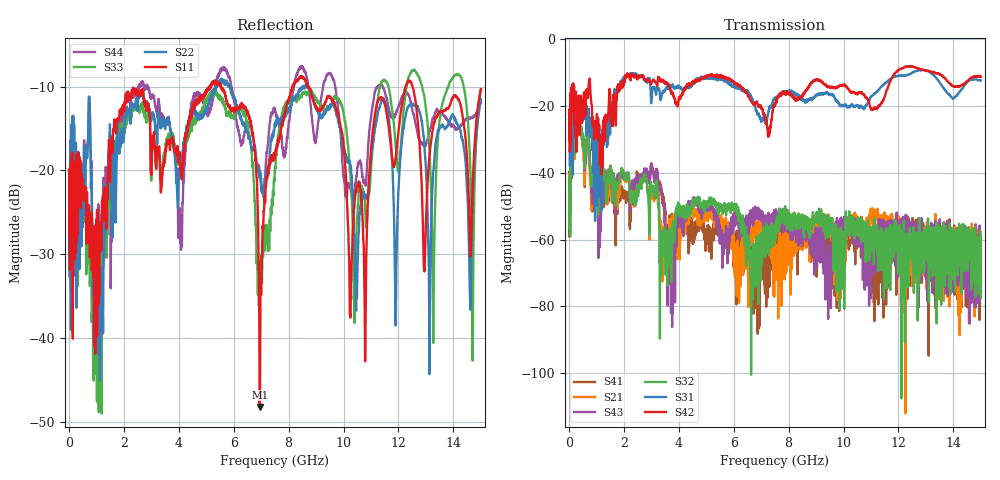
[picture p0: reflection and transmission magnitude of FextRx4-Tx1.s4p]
!  = SDD11
!  = SDD12
!  = SDC11
!  = SDC12
!  = SDD21
!  = SDD22
!  = SDC21
!  = SDC22
!  = SCD11
!  = SCD12
!  = SCC11
!  = SCC12
!  = SCD21
!  = SCD22
!  = SCC21
!  = SCC22
! FILE: N:\QM 2007\Prüfprotokolle\Highspeed\Konfektionierte Ltg\L45593-D106\D30\8216\0002\Fext\FextRx4-Tx1.s4p
# MHz S DB R 50.00
! FREQ  S11  S12  S13  S14
!  S21  S22  S23  S24
!  S31  S32  S33  S34
!  S41  S42  S43  S44
!  DB  ANG  DB  ANG  DB  ANG  DB  ANG
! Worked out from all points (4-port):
!   2999 points, 10 MHz to 15 GHz, reference 50 ohm
!   strongest paths, dB at 10 MHz, 3.755 GHz, 7.505 GHz, 11.26 GHz, 15 GHz:
!     S42: -24.0, -15.6, -19.8, -20.3, -11.3
!     S31: -24.8, -13.8, -17.9, -15.3, -12.3
!     S32: -41.6, -60.8, -56.9, -58.5, -77.6
!     S43: -51.1, -65.0, -53.2, -63.2, -77.1
!     S21: -42.3, -54.2, -63.5, -56.0, -69.0
!     S41: -39.7, -56.6, -57.4, -67.7, -60.1
!   lowest |S11| = -48.2 dB at 6.955 GHz (marker M1), VSWR 1.01, Z = 50.2 - j0.357 ohm
!   |S11| at or under -10 dB: start of sweep to 5.122 GHz; 5.536 GHz to 8.15 GHz (2.614 GHz wide, 38.2 % of centre); 8.719 GHz to 12.26 GHz (3.541 GHz wide, 33.8 % of centre)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
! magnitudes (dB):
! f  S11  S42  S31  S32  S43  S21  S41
! 10 MHz  -19.9  -24.0  -24.8  -41.6  -51.1  -42.3  -39.7
! 355 MHz  -20.2  -21.8  -20.6  -27.2  -27.7  -28.2  -28.0
! 3.73 GHz  -16.3  -16.2  -14.0  -62.7  -76.3  -57.1  -54.6
! 6.955 GHz  -48.2  -19.8  -23.6  -71.3  -53.5  -59.0  -66.8
! 8.28 GHz  -9.3  -17.8  -16.7  -55.1  -60.6  -56.6  -57.2
! 10.78 GHz  -40.5  -17.0  -20.4  -55.6  -64.6  -54.9  -56.6
! 15 GHz  -10.3  -11.3  -12.3  -77.6  -77.1  -69.0  -60.1
